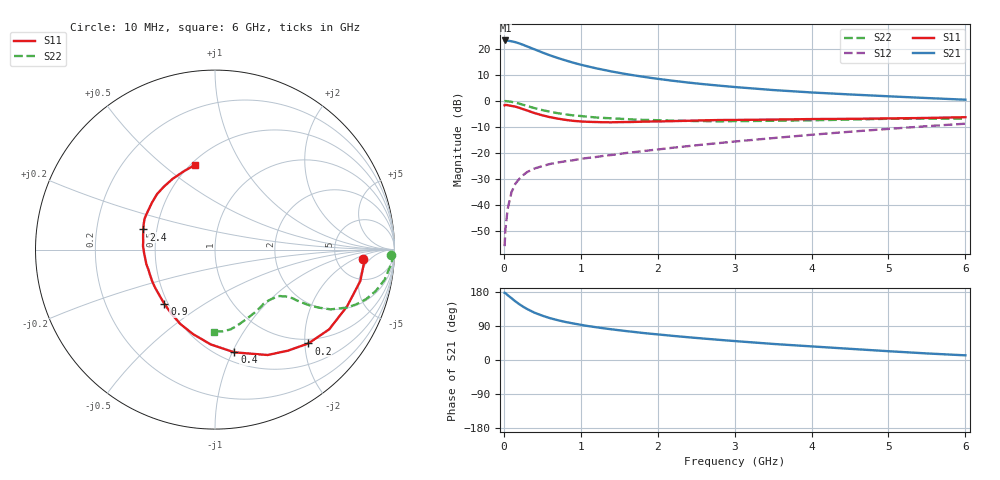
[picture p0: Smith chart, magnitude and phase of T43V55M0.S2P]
! Infineon Technologies  Discrete & RF Semiconductors
! BFR182T
! Si NPN RF Bipolar Junction Transistor in SC75
! VCE = 3.5 V  IC = 5 mA
! Common Emitter S-Parameters:  October  1999
# GHz  S  MA  R  50
!  f  S11  S21  S12  S22
! GHz  MAG  ANG  MAG  ANG  MAG  ANG  MAG  ANG
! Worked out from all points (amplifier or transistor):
!   36 points, 10 MHz to 6 GHz, reference 50 ohm
!   highest |S21| = 23.3 dB at 20 MHz (marker M1)
!   |S21| within 3 dB of that: start of sweep to 362.8 MHz
!   unconditionally stable (mu >= 1): 1.397 GHz to 4.023 GHz
!   at 250 MHz: K = 0.29, MSG = 25.1 dB, |S12| = -28.6 dB
!   at 1.4 GHz: K = 1.00, MAG = 15.9 dB, |S12| = -20.8 dB
!   at 6 GHz: K = 0.84, MSG = 4.6 dB, |S12| = -8.8 dB
!   lowest NFmin = 1.20 dB at 450 MHz
!   S11 on the Smith chart (normalised r, x): 10 MHz: 9.42, -2.95; 200 MHz: 0.91, -2.08; 400 MHz: 0.59, -1.02; 900 MHz: 0.48, -0.35; 2.4 GHz: 0.42, +0.11; 6 GHz: 0.53, +0.65
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0.01  0.8238 -3.5  14.53 177.4  0.0016 78.6  0.9825 -1.8
0.02  0.8367 -3.5  14.58 176.6  0.0033 91.3  0.9951 -2.1
0.05  0.8283 -12.2  14.48 171.1  0.0084 84.9  0.9821 -5.2
0.1  0.801 -23.2  14.03 163.0  0.0176 79.0  0.9598 -10.1
0.15  0.776 -34.9  13.51 154.7  0.0255 72.8  0.9249 -14.4
0.2  0.7377 -45.1  12.81 147.4  0.0314 69.6  0.8866 -18.1
0.25  0.6944 -54.2  12.01 140.8  0.0372 64.1  0.8436 -21.2
0.3  0.6562 -63.5  11.23 134.8  0.0425 61.9  0.8034 -23.7
0.4  0.5826 -79.3  9.818 124.7  0.0501 57.0  0.7258 -27.3
0.5  0.5288 -92.6  8.561 117.0  0.0556 54.1  0.6662 -29.1
0.6  0.4864 -104.6  7.534 110.4  0.0611 52.6  0.6189 -30.4
0.7  0.4566 -115.3  6.711 105.1  0.0651 52.5  0.5806 -31.1
0.9  0.4138 -132.9  5.452 96.5  0.0721 52.3  0.527 -32.0
1.1  0.3957 -147.1  4.59 89.4  0.0802 53.3  0.4946 -32.7
1.3  0.3883 -158.9  3.957 83.6  0.0879 54.9  0.4701 -33.7
1.6  0.3917 -172.6  3.264 76.1  0.0999 56.9  0.4455 -35.5
2.2  0.4083 168.9  2.44 63.6  0.1258 59.9  0.4181 -41.3
2.4  0.4149 164.3  2.253 60.0  0.1351 60.5  0.4114 -43.7
3.5  0.4375 143.6  1.619 42.4  0.1925 61.4  0.4145 -57.6
4.5  0.4518 129.0  1.332 29.5  0.2552 58.9  0.4369 -71.9
5.5  0.4702 111.4  1.136 17.3  0.3264 54.5  0.4575 -84.8
6  0.4855 103.0  1.055 12.3  0.3644 51.1  0.4564 -90.4
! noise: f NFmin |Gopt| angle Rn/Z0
0.45  1.2  0.27  37  0.3
0.9  1.3  0.25  75  0.23
1.8  1.9  0.21  145  0.2
